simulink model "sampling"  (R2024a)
settings: Solver=ode45  StartTime=0.0  StopTime=0.01  MaxStep=1e-6  RelTol=1e-4  EnableMultiTasking=on

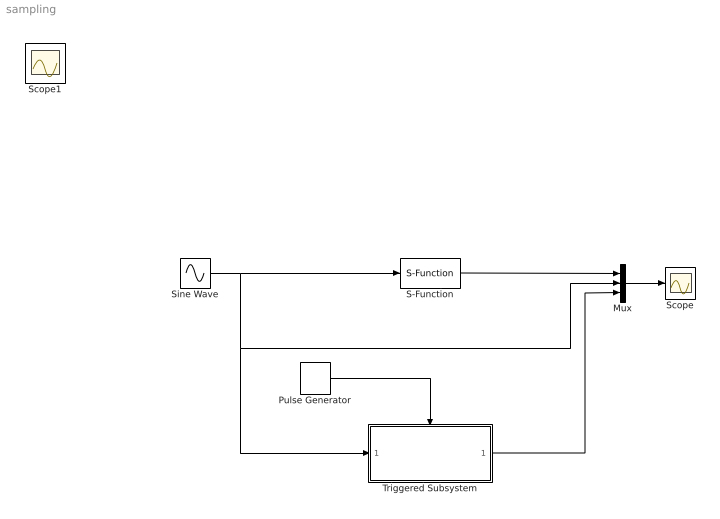
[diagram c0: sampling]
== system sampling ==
  Mux : Mux  Inputs=3
  Pulse Generator : DiscretePulseGenerator  PulseType=Time based  Period=1/1000  PulseWidth=50
  S-Function : S-Function  FunctionName=controller  SFunctionDeploymentMode=off  EnableBusSupport=off
  Scope : Scope
  Sine Wave : Sin  Frequency=2*pi*100  SampleTime=0
  Triggered Subsystem : Subsystem  TreatAsAtomicUnit=on
  Scope1 : Scope
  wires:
  Sine Wave/1 -> S-Function/1, Mux/2, Triggered Subsystem/1(In1)
  S-Function/1 -> Mux/1
  Mux/1 -> Scope/1
  Triggered Subsystem/1(Out1) -> Mux/3
  Pulse Generator/1 -> Triggered Subsystem/Trigger

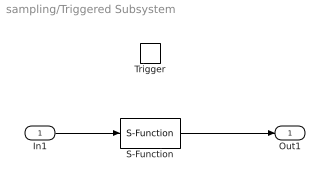
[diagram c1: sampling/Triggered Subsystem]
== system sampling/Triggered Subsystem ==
  In1 : Inport
  Trigger : TriggerPort  VariantControl=(inherit)
  S-Function : S-Function  FunctionName=controller  SFunctionDeploymentMode=off  EnableBusSupport=off
  Out1 : Outport
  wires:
  In1/1 -> S-Function/1
  S-Function/1 -> Out1/1
